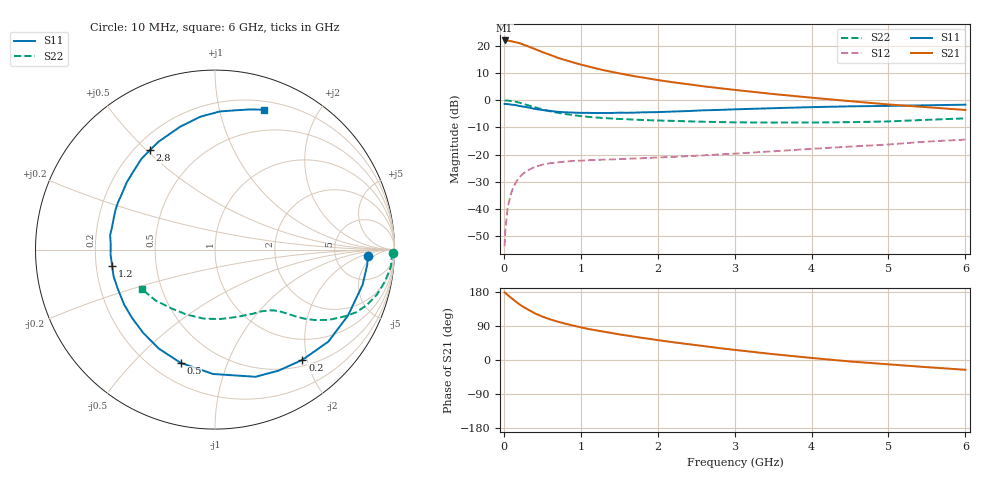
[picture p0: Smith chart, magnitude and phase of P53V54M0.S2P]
! SIEMENS Small Signal Semiconductors
! BFP183
! Si NPN RF Bipolar Junction Transistor in SOT143
! VCE = 3.5 V  IC = 4 mA
! Common Emitter S-Parameters:  March  1996
# GHz  S  MA  R  50
!  f  S11  S21  S12  S22
! GHz  MAG  ANG  MAG  ANG  MAG  ANG  MAG  ANG
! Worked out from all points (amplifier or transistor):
!   36 points, 10 MHz to 6 GHz, reference 50 ohm
!   highest |S21| = 21.9 dB at 10 MHz (marker M1)
!   |S21| within 3 dB of that: start of sweep to 390.6 MHz
!   unconditionally stable (mu >= 1): 1.695 GHz to 5.693 GHz
!   at 250 MHz: K = 0.18, MSG = 23.7 dB, |S12| = -27.0 dB
!   at 1.4 GHz: K = 0.87, MSG = 16.1 dB, |S12| = -21.7 dB
!   at 6 GHz: K = 0.95, MSG = 5.4 dB, |S12| = -14.5 dB
!   S11 on the Smith chart (normalised r, x): 10 MHz: 12, -3; 200 MHz: 0.60, -1.92; 500 MHz: 0.31, -0.70; 1.2 GHz: 0.27, -0.07; 2.8 GHz: 0.26, +0.51; 6 GHz: 0.28, +1.37
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0.01  0.8507 -2.5  12.44 178.5  0.0021 84.0  0.9946 -1.1
0.02  0.8529 -5.5  12.42 177.1  0.0042 80.6  0.9858 -2.2
0.05  0.8454 -13.4  12.37 171.4  0.0109 84.1  0.9851 -5.4
0.1  0.827 -26.4  12.01 163.1  0.0207 75.6  0.9626 -10.8
0.15  0.8134 -39.1  11.57 155.0  0.03 70.0  0.9361 -15.6
0.2  0.7839 -51.6  11.16 147.3  0.0383 64.3  0.9002 -20.1
0.25  0.7616 -62.3  10.49 140.4  0.0446 58.4  0.8598 -24.0
0.3  0.7438 -72.3  9.874 134.8  0.0507 54.0  0.8168 -27.0
0.4  0.6931 -90.9  8.705 123.5  0.0595 46.7  0.7438 -31.8
0.5  0.6595 -106.8  7.618 114.6  0.0654 40.8  0.6787 -35.3
0.6  0.6345 -119.4  6.788 107.4  0.0696 36.6  0.6269 -37.8
0.7  0.6128 -130.7  5.986 101.3  0.0724 33.5  0.5867 -39.5
0.8  0.5989 -140.5  5.426 95.7  0.0747 31.1  0.5566 -40.7
1.1  0.5846 -165.1  4.149 81.9  0.0791 27.0  0.4936 -43.9
1.2  0.5802 -171.1  3.82 78.3  0.0799 26.1  0.4815 -45.1
1.6  0.5873 167.1  2.917 64.5  0.0842 25.2  0.4469 -49.5
2.2  0.6185 142.6  2.127 46.9  0.0911 26.2  0.4166 -58.6
2.8  0.6623 123.1  1.662 31.4  0.101 27.7  0.3963 -70.0
3.5  0.7119 105.8  1.297 15.5  0.1153 28.4  0.3881 -85.7
4.5  0.7701 88.0  0.959 -3.9  0.1406 26.3  0.395 -113.3
5.5  0.8049 76.0  0.743 -18.9  0.174 22.5  0.4359 -139.4
6  0.8262 70.6  0.661 -25.8  0.1891 18.5  0.4636 -151.7
